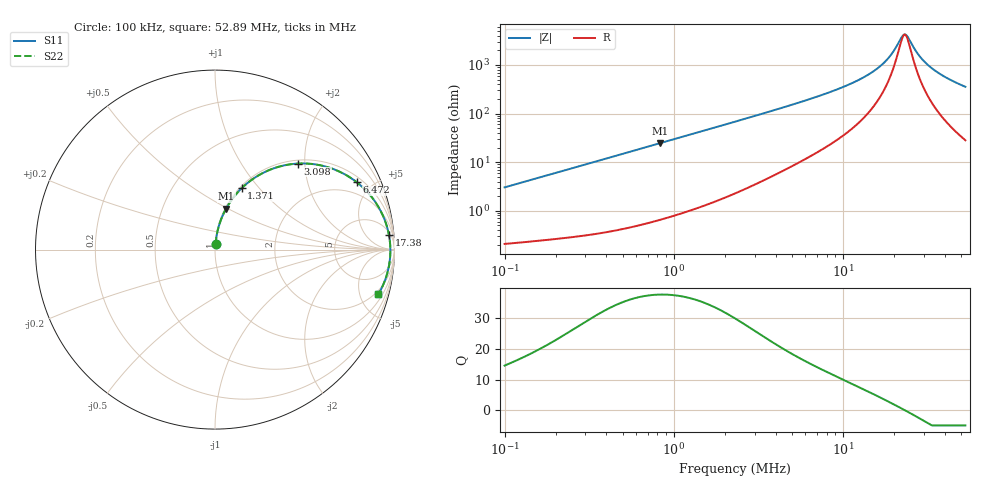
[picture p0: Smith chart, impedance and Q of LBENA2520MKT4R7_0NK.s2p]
! LBENA2520MKT4R7_0NK  S-PARAMETER MODEL  ( General Type )
! Model Generated by TAIYO YUDEN Corporation (http://www.ty-top.com)
! Version 1.0
! TAIYO YUDEN Control No. 211116
! Copyright(c) 2021 TAIYO YUDEN CO.,LTD. All Rights Reserved.
! Product Description (link to TY-COMPAS)
! https://ds.yuden.co.jp/TYCOMPAS/or/detail?pn=LBENA2520MKT4R7M0NK&u=M
! Products Name : Inductors
! Characteristics :
!  Inductance : 4.7 uH , SRF(min) : -Hz , DC Resistance(max) : 0.185 Ohm
!  Rated Current : Saturation :2100 mA , Temp Rise : 1500 mA
!  Case Size : 2.5 x 2.0 / 0.098 x 0.079 [mm/inch] , Thickness : 1.2 / 0.047 [mm/inch]
!  (Conditions: Temperature = 25 degC , DC Bias Current/Voltage = 0A / 0V)
! External Node Assignments :
!  1  o---GGG---o  2
! GND o---------o GND
! Frequency Range : 0.1MHz  -  52.890102MHz  [ 402 STEP ]
# MHz S RI R 50
! Freq[MHz].  S11 Real  S11 Imag  S21 Real  S21 Imag  S12 Real  S12 Imag  S22 Real  S22 Imag
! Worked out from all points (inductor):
!   401 points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, 100 kHz to 52.89 MHz, reference 50 ohm
!   read as one part in series: L = 4.79 uH near 103.2 kHz
!   highest Q = 37.8 at 830.1 kHz (marker M1), where L = 4.71 uH
!   self-resonance near 23.17 MHz
!   S11 on the Smith chart (normalised r, x): 100 kHz: 1.00, +0.06; 1.371 MHz: 1.02, +0.81; 3.098 MHz: 1.07, +1.84; 6.472 MHz: 1.27, +4.05; 17.38 MHz: 7, +21; 52.89 MHz: 1.56, -7.10
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0.1  0.00298 0.0301  0.997 -0.0301  0.997 -0.0301  0.00298 0.0301
0.285868  0.0102 0.0842  0.9898 -0.0842  0.9898 -0.0842  0.0102 0.0842
0.817204  0.0607 0.2258  0.9393 -0.2258  0.9393 -0.2258  0.0607 0.2258
0.830116  0.0624 0.2289  0.9376 -0.2289  0.9376 -0.2289  0.0624 0.2289
1.37091  0.1478 0.3412  0.8522 -0.3412  0.8522 -0.3412  0.1478 0.3412
2.299785  0.3222 0.451  0.6778 -0.451  0.6778 -0.451  0.3222 0.451
3.097758  0.4609 0.4792  0.5391 -0.4792  0.5391 -0.4792  0.4609 0.4792
4.37354  0.6291 0.459  0.3709 -0.459  0.3709 -0.459  0.6291 0.459
6.472082  0.7894 0.3759  0.2106 -0.3759  0.2106 -0.3759  0.7894 0.3759
6.574344  0.7947 0.3717  0.2053 -0.3717  0.2053 -0.3717  0.7947 0.3717
9.137546  0.8856 0.2761  0.1144 -0.2761  0.1144 -0.2761  0.8856 0.2761
11.92815  0.933 0.1951  0.067 -0.1951  0.067 -0.1951  0.933 0.1951
14.85563  0.9578 0.1293  0.0422 -0.1293  0.0422 -0.1293  0.9578 0.1293
17.37703  0.9689 0.0833  0.0311 -0.0833  0.0311 -0.0833  0.9689 0.0833
18.79393  0.9726 0.0605  0.0274 -0.0605  0.0274 -0.0605  0.9726 0.0605
22.33112  0.9769 0.0106  0.0231 -0.0106  0.0231 -0.0106  0.9769 0.0106
23.40646  0.9771 -0.00297  0.0229 0.00297  0.0229 0.00297  0.9771 -0.00297
24.15197  0.9771 -0.012  0.0229 0.012  0.0229 0.012  0.9771 -0.012
28.2512  0.9742 -0.0576  0.0258 0.0576  0.0258 0.0576  0.9742 -0.0576
32.53216  0.9676 -0.0993  0.0324 0.0993  0.0324 0.0993  0.9676 -0.0993
40.51641  0.9491 -0.1657  0.0509 0.1657  0.0509 0.1657  0.9491 -0.1657
52.8901  0.91 -0.2492  0.09 0.2492  0.09 0.2492  0.91 -0.2492
